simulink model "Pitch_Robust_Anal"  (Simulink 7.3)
settings: Solver=ode45  StartTime=0.0  StopTime=44  RelTol=1e-3
InitFcn:
  | init
undefined symbols (not defined in the file or in its folder): Apu, Bpu, Cpu, Dpu, Kmix, Kq

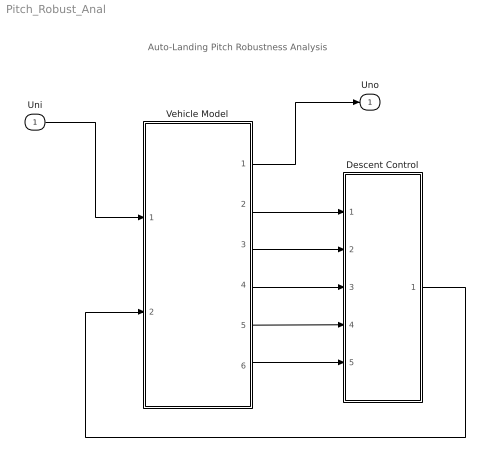
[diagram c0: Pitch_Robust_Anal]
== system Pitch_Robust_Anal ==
  note: Auto-Landing Pitch Robustness Analysis
  Uni : Inport  OutDataType=sfix(16)  OutScaling=2^0
  Descent Control : Subsystem
  Vehicle Model : Subsystem
  Uno : Outport  OutDataType=sfix(16)  OutScaling=2^0
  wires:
  Vehicle Model/2(theta) -> Descent Control/1(theta)
  Vehicle Model/3(q) -> Descent Control/2(q)
  Vehicle Model/4(dH) -> Descent Control/3(dH)
  Vehicle Model/5(dV) -> Descent Control/4(dV)
  Vehicle Model/6(Nz) -> Descent Control/5(Nz)
  Descent Control/1((dQ,dV)) -> Vehicle Model/2("(dQ, dV)")
  Vehicle Model/1(Uno) -> Uno/1
  Uni/1 -> Vehicle Model/1(Uni)

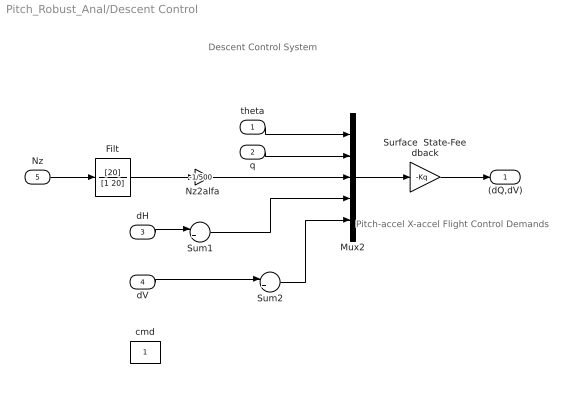
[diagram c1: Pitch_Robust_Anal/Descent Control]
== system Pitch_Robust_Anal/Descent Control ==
  note: Descent Control System
  note: Pitch-accel X-accel Flight Control Demands
  theta : Inport
  q : Inport  Port=2
  dH : Inport  Port=3
  dV : Inport  Port=4
  Nz : Inport  Port=5
  Filt : TransferFcn  Numerator=[20]  Denominator=[1 20]
  Mux2 : Mux  Inputs=5
  Nz2alfa : Gain  Gain=-1/500  ParameterDataType=sfix(16)  ParameterScaling=2^0  OutDataType=sfix(16)  OutScaling=2^0
  Sum1 : Sum  Inputs=|+-  OutDataType=sfix(16)  OutScaling=2^0
  Sum2 : Sum  Inputs=|+-  OutDataType=sfix(16)  OutScaling=2^0
  Surface  State-Feedback : Gain  Gain=-Kq  Multiplication=Matrix(K*u)  ParameterDataType=sfix(16)  ParameterScaling=2^0  OutDataType=sfix(16)  OutScaling=2^0
  cmd : Constant  OutDataType=fixdt(1, 16)  OutScaling=2^0
  (dQ,dV) : Outport
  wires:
  Filt/1 -> Nz2alfa/1
  Nz2alfa/1 -> Mux2/3
  Surface  State-Feedback/1 -> (dQ,dV)/1
  Mux2/1 -> Surface  State-Feedback/1
  Nz/1 -> Filt/1
  q/1 -> Mux2/2
  theta/1 -> Mux2/1
  dH/1 -> Sum1/1
  Sum1/1 -> Mux2/4
  Sum2/1 -> Mux2/5
  dV/1 -> Sum2/1

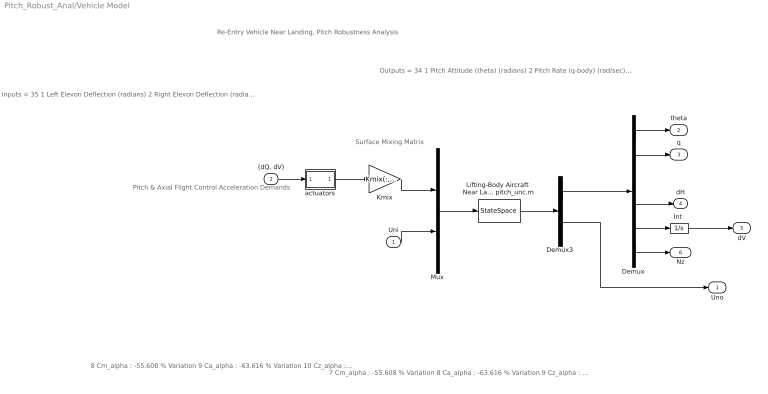
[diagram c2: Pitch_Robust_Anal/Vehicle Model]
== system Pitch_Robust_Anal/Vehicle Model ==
  note: Re-Entry Vehicle Near Landing, Pitch Robustness Analysis
  note: Surface Mixing Matrix
  note: Pitch & Axial Flight Control Acceleration Demands
  note: Outputs = 34 1 Pitch Attitude (theta) (radians) 2 Pitch Rate (q-body) (rad/sec) 3 Angle of attack, alfa, (radians) 4 Change in Altitude, delta-h, (feet) 5 Forward Accelerat (V-dot) (ft/sec) 6 Accelerom #3, (along Z), (ft/sec^2)
  note: Inputs = 35 1 Left Elevon Deflection (radians) 2 Right Elevon Deflection (radians) 3 Vertical Rudder Deflection (radians) 4 Upper Left Body-Flap Deflection (radians) 5 Upper Right Body-Flap Deflection (radians) 6 Lower Left Body-Flap Deflection (radians) 7 Lower Right Body-Flap Deflection (radians)
  note: 8 Cm_alpha : -55.608 % Variation 9 Ca_alpha : -63.616 % Variation 10 Cz_alpha : -20.621 % Variation 11 Cm_0 : -75.382 % Variation 12 CZ_0 : -10.833 % Variation 13 Cm_q : -52.604 % Variation 14 CA_0 : 71.590 % Variation 15 I_yy : 4.619 % Variation 16 Xcg locat: -2.934 % Variation 17 Xcg locat: -2.934 % Variation 18 Ca_surf 1: -148.128 % Variation 19 Cz_surf 1: -86.207 % Variation 20 Cm_surf 1: -55.746 % Variation 21 Ca_surf 2: -148.128 % Variation 22 Cz_surf 2: -86.207 % Variation 23 Cm_surf 2: -55.746 % Variation 24 Ca_surf 4: -109.953 % Variation 25 Cz_surf 4: -43.471 % Variation 26 Cm_surf 4: -157.762 % Variation 27 Ca_surf 5: -109.953 % Variation 28 Cz_surf 5: -43.471 % Variation 29 Cm_surf 5: -157.762 % Variation 30 Ca_surf 6: 44.037 % Variation 31 Cz_surf 6: -38.604 % Variation 32 Cm_surf 6: -53.298 % Variation 33 Ca_surf 7: 44.037 % Variation 34 Cz_surf 7: -38.604 % Variation 35 Cm_surf 7: -53.298 % Variation
  note: 7 Cm_alpha : -55.608 % Variation 8 Ca_alpha : -63.616 % Variation 9 Cz_alpha : -20.621 % Variation 10 Cm_0 : -75.382 % Variation 11 CZ_0 : -10.833 % Variation 12 Cm_q : -52.604 % Variation 13 CA_0 : 71.590 % Variation 14 I_yy : 4.619 % Variation 15 Xcg locat: -2.934 % Variation 16 Xcg locat: -2.934 % Variation 17 Ca_surf 1: -148.128 % Variation 18 Cz_surf 1: -86.207 % Variation 19 Cm_surf 1: -55.746 % Variation 20 Ca_surf 2: -148.128 % Variation 21 Cz_surf 2: -86.207 % Variation 22 Cm_surf 2: -55.746 % Variation 23 Ca_surf 4: -109.953 % Variation 24 Cz_surf 4: -43.471 % Variation 25 Cm_surf 4: -157.762 % Variation 26 Ca_surf 5: -109.953 % Variation 27 Cz_surf 5: -43.471 % Variation 28 Cm_surf 5: -157.762 % Variation 29 Ca_surf 6: 44.037 % Variation 30 Cz_surf 6: -38.604 % Variation 31 Cm_surf 6: -53.298 % Variation 32 Ca_surf 7: 44.037 % Variation 33 Cz_surf 7: -38.604 % Variation 34 Cm_surf 7: -53.298 % Variation
  Uni : Inport  OutDataType=sfix(16)  OutScaling=2^0
  "(dQ, dV)" : Inport  Port=2  OutDataType=sfix(16)  OutScaling=2^0
  Demux : Demux  Outputs=6
  Demux3 : Demux  Outputs=[6, 28]
  "Int " : Integrator
  Kmix : Gain  Gain=Kmix(:,[2,4])  Multiplication=Matrix(K*u)  ParameterDataType=sfix(16)  ParameterScaling=2^0  OutDataType=sfix(16)  OutScaling=2^0
  "Lifting-Body Aircraft  Near Landing,  Pitch Robust Analysis  (28 Uncs)  from file pitch_unc.m" : StateSpace  A=Apu  B=Bpu  C=Cpu  D=Dpu
  Mux : Mux  Inputs=[7, 28]
  actuators : Subsystem
  Uno : Outport  OutDataType=sfix(16)  OutScaling=2^0
  theta : Outport  Port=2  OutDataType=sfix(16)  OutScaling=2^0
  q : Outport  Port=3  OutDataType=sfix(16)  OutScaling=2^0
  dH : Outport  Port=4  OutDataType=sfix(16)  OutScaling=2^0
  dV : Outport  Port=5  OutDataType=sfix(16)  OutScaling=2^0
  Nz : Outport  Port=6  OutDataType=sfix(16)  OutScaling=2^0
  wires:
  Mux/1 -> "Lifting-Body Aircraft  Near Landing,  Pitch Robust Analysis  (28 Uncs)  from file pitch_unc.m"/1
  Kmix/1 -> Mux/1
  "(dQ, dV)"/1 -> actuators/1(In)
  Uni/1 -> Mux/2
  "Lifting-Body Aircraft  Near Landing,  Pitch Robust Analysis  (28 Uncs)  from file pitch_unc.m"/1 -> Demux3/1
  Demux3/1 -> Demux/1
  Demux3/2 -> Uno/1
  actuators/1(out) -> Kmix/1
  "Int "/1 -> dV/1
  Demux/1 -> theta/1
  Demux/2 -> q/1
  Demux/4 -> dH/1
  Demux/5 -> "Int "/1
  Demux/6 -> Nz/1

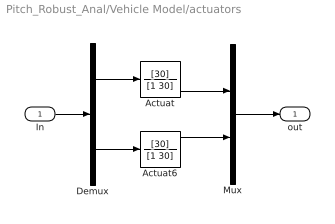
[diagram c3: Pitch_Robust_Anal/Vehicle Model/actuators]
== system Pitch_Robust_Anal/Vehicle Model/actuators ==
  In : Inport
  Actuat : TransferFcn  Numerator=[30]  Denominator=[1 30]
  Actuat6 : TransferFcn  Numerator=[30]  Denominator=[1 30]
  Demux : Demux  Outputs=2
  Mux : Mux  Inputs=2
  out : Outport
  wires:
  Actuat6/1 -> Mux/2
  Actuat/1 -> Mux/1
  Demux/2 -> Actuat6/1
  Demux/1 -> Actuat/1
  Mux/1 -> out/1
  In/1 -> Demux/1
